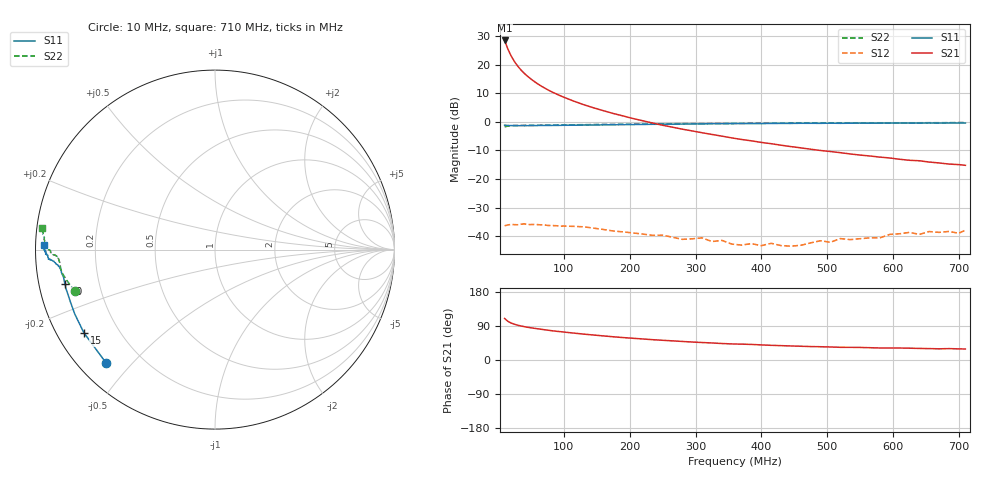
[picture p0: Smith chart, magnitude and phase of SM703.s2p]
!  POLYFET RF DEVICES
!  S PARAMETERS FOR
!  SM703
!  VDS=28, IDQ=600MA
# MHZ  S  MA  R  50.0000
! SCATTERING PARAMETERS :
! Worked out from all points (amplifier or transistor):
!   60 points, 10 MHz to 710 MHz, reference 50 ohm
!   highest |S21| = 28.5 dB at 10 MHz (marker M1)
!   |S21| within 3 dB of that: start of sweep to 14.96 MHz
!   unconditionally stable (mu >= 1): 273.4 MHz to 294.6 MHz; 295.2 MHz to end of sweep
!   at 60 MHz: K = 0.17, MSG = 24.6 dB, |S12| = -36.0 dB
!   at 280 MHz: K = 1.06, MAG = 17.7 dB, |S12| = -41.1 dB
!   at 710 MHz: K = 1.43, MAG = 7.4 dB, |S12| = -37.9 dB
!   S11 on the Smith chart (normalised r, x): 10 MHz: 0.08, -0.43; 15 MHz: 0.08, -0.29; 40 MHz: 0.08, -0.11; 710 MHz: 0.02, +0.01
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10  0.876 -133.7  26.51 109.5  0.01522 19.5  0.8158 -163.5
15  0.8652 -147.5  18.72 102.1  0.01575 14.6  0.844 -168.4
20  0.8599 -155.3  14.14 97.5  0.01603 7.6  0.8599 -171.1
25  0.8567 -159.9  11.3 94.3  0.01591 5.6  0.8658 -172.7
30  0.8564 -163.1  9.405 91.8  0.01585 5.5  0.8667 -173.9
35  0.8584 -165.4  8.042 89.7  0.0162 3.4  0.8674 -174.7
40  0.8569 -167.0  7.032 88.0  0.01643 3.4  0.8681 -175.4
45  0.8581 -168.3  6.24 86.3  0.01595 -0.2  0.8707 -175.6
50  0.8572 -169.2  5.612 84.9  0.01599 -2.8  0.8712 -176.1
55  0.8585 -169.9  5.087 83.6  0.01603 -2.6  0.8711 -176.3
65  0.8639 -171.2  4.269 81.2  0.01579 -1.2  0.8753 -176.9
75  0.8645 -172.0  3.668 78.8  0.01544 -4.3  0.8783 -176.9
85  0.867 -172.7  3.211 76.5  0.01531 -4.5  0.88 -177.5
100  0.8709 -173.2  2.692 73.7  0.01506 -4.8  0.8839 -177.6
130  0.8786 -174.1  1.997 68.3  0.0146 -9.8  0.8926 -178.1
175  0.89 -174.9  1.401 61.3  0.01233 -9.2  0.9023 -178.4
250  0.9089 -176.2  0.8713 52.0  0.01042 -0.5  0.9225 -180.0
370  0.9325 -177.6  0.4915 41.8  0.00699 17.0  0.9402 178.0
445  0.939 -178.7  0.369 37.1  0.00669 37.7  0.9506 177.1
490  0.9417 -178.9  0.3155 35.0  0.00833 52.0  0.9532 176.2
595  0.9521 179.7  0.2334 31.6  0.01074 68.1  0.9615 174.6
710  0.9542 178.5  0.1736 29.1  0.01276 73.6  0.9725 172.9
